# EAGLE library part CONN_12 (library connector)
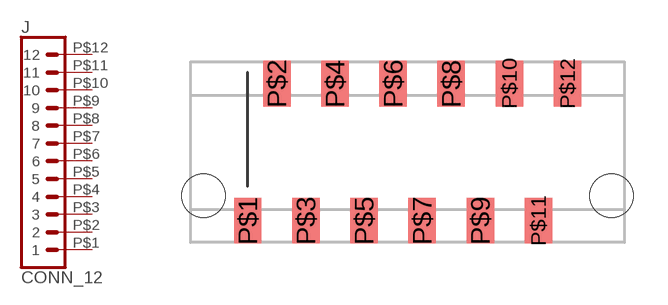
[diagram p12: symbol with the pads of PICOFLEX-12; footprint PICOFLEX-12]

Designator prefix J

## CONN_12PICOFLEX  [PICOFLEX-12]
P$1  1  pas
P$2  2  pas
P$3  3  pas
P$4  4  pas
P$5  5  pas
P$6  6  pas
P$7  7  pas
P$8  8  pas
P$9  9  pas
P$10  10  pas
P$11  11  pas
P$12  12  pas

## Footprint PICOFLEX-12 (pad centres in mm)
smd 1.2 x 2: P$1 0,0; P$2 1.27,6; P$3 2.54,0; P$4 3.81,6; P$5 5.08,0; P$6 6.35,6; P$7 7.62,0; P$8 8.89,6; P$9 10.16,0; P$10 11.43,6; P$11 12.7,0; P$12 13.97,6
hole 1.9 at -1.93,1.1
hole 1.9 at 15.89,1.1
